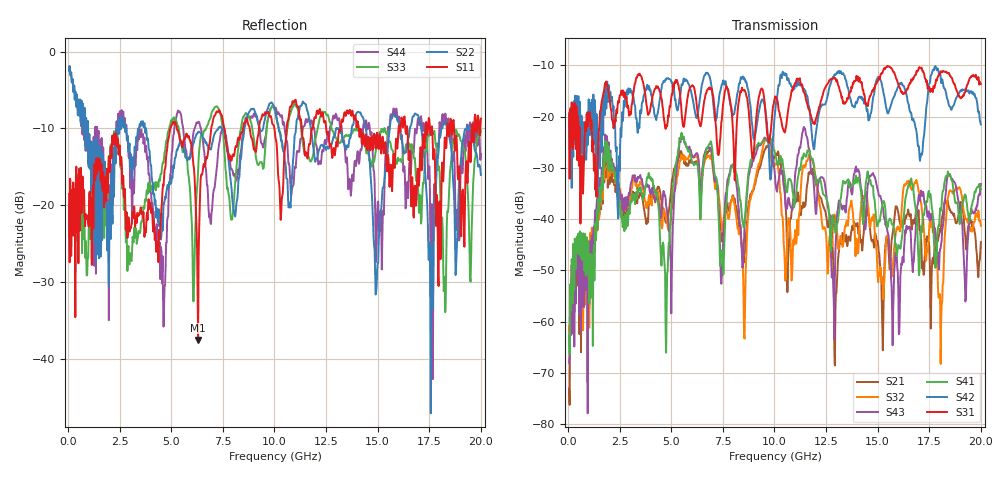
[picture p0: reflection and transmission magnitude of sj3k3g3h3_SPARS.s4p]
! FILE: E:\users\goganessyan\GBX_Backplane\FR408_backplane\1m_INBOUND_NEXT\sj3k3g3h3_SPARS.s4p
# MHZ S RI R 50.00
! FREQ  S11  S12  S13  S14
!  S21  S22  S23  S24
!  S31  S32  S33  S34
!  S41  S42  S43  S44
!  REAL  IMAG  REAL  IMAG  REAL  IMAG  REAL  IMAG
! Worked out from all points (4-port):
!   799 points, 50 MHz to 20 GHz, reference 50 ohm
!   strongest paths, dB at 50 MHz, 5.025 GHz, 10.03 GHz, 15.03 GHz, 20 GHz:
!     S31: -19.6, -15.6, -16.1, -12.9, -13.6
!     S42: -19.2, -13.4, -19.3, -12.3, -21.5
!     S41: -62.7, -36.6, -27.1, -40.9, -34.2
!     S43: -68.0, -50.7, -31.6, -34.6, -33.2
!     S32: -60.9, -37.5, -29.2, -52.3, -41.3
!     S21: -73.0, -32.6, -27.8, -45.1, -44.5
!   lowest |S11| = -37.5 dB at 6.3 GHz (marker M1), VSWR 1.03, Z = 48.8 - j0.482 ohm
!   |S11| at or under -10 dB: start of sweep to 4.956 GHz; 5.266 GHz to 6.937 GHz (1.671 GHz wide, 27.4 % of centre); 14.09 GHz to 16.01 GHz (1.926 GHz wide, 12.8 % of centre)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
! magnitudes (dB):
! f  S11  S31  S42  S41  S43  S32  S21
! 50 MHz  -18.5  -19.6  -19.2  -62.7  -68.0  -60.9  -73.0
! 1.825 GHz  -18.6  -13.5  -13.6  -26.7  -25.5  -28.1  -29.3
! 4.75 GHz  -13.7  -22.2  -12.8  -66.1  -37.3  -39.5  -40.7
! 6.3 GHz  -37.5  -20.0  -19.1  -30.2  -27.7  -28.7  -29.8
! 8.525 GHz  -9.3  -15.0  -12.7  -41.6  -44.0  -62.6  -48.3
! 16.05 GHz  -9.9  -14.2  -13.7  -45.5  -62.2  -41.8  -40.2
! 20 GHz  -8.7  -13.6  -21.5  -34.2  -33.2  -41.3  -44.5
